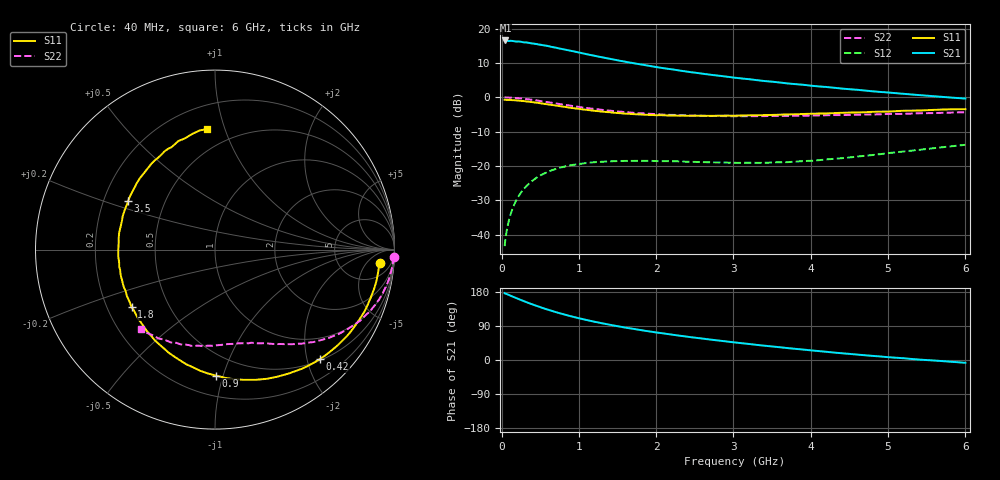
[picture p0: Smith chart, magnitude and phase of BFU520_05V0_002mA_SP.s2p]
! Filename:  P:\Prog\Test\Noise\ATS_data\Testdata_Net\03 Spar\BFU520_APG2013_37_A05_05p0V_002mA_SP_CM01_D.s2p
! Date/Time: Fri 26/Apr/2013 13:00:07
! BFU520_APG2013_37_A05_05p0V_1to20mA_SP_CM01_Bias2_R.s2p
! MDIF S-parameter v. bias file
! BFU520_APG2013_37_A05_05p0V_1to20mA_SP_CM01
! Date/time Tue Apr 23 15:26:19 2013
! VAR V_out= 5.0000
! VAR I_out= 1.9950
! VAR V_in= 0.8075
! VAR I_in= 0.0222
! Device data file deembeded for feedlines and parallel
! Original file: \03 Spar\BFU520_APG2013_37_A05_05p0V_002mA_SP_CM01_R.s2p
! Feed-files: PR047V01_250413_Feed1.s2p, PR047V01_250413_Feed2.s2p
! Parallel-file: PR047V01_250413_Par.s2p
# MHz S MA R 50
!  Freq-MHz  S11-mag  S11-arg  S21-mag  S21-arg  S12-mag  S12-arg  S22-mag  S22-arg
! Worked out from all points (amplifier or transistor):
!   98 points, 40 MHz to 6 GHz, reference 50 ohm
!   highest |S21| = 16.5 dB at 50 MHz (marker M1)
!   |S21| within 3 dB of that: start of sweep to 894.5 MHz
!   unconditionally stable (mu >= 1): 2.993 GHz to 4.97 GHz
!   at 300 MHz: K = 0.11, MSG = 21.2 dB, |S12| = -26.4 dB
!   at 1.6 GHz: K = 0.53, MSG = 14.4 dB, |S12| = -18.5 dB
!   at 6 GHz: K = 0.83, MSG = 6.7 dB, |S12| = -13.8 dB
!   S11 on the Smith chart (normalised r, x): 40 MHz: 13, -12; 420 MHz: 0.53, -2.25; 900 MHz: 0.34, -0.95; 1.8 GHz: 0.30, -0.29; 3.5 GHz: 0.30, +0.24; 6 GHz: 0.36, +0.87
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40  0.9211 -4.6  6.69 176.6  0.006855 86.6  0.996 -2.4
50  0.9193 -5.7  6.709 175.0  0.008572 86.3  0.9963 -2.9
100  0.916 -11.2  6.587 171.2  0.01699 82.9  0.9909 -6.1
120  0.9133 -13.6  6.634 169.4  0.0203 81.6  0.9881 -7.3
180  0.904 -20.3  6.494 164.4  0.03012 77.4  0.979 -11.0
220  0.8961 -24.8  6.479 160.9  0.03632 74.8  0.9696 -13.4
320  0.8721 -35.7  6.284 152.8  0.05091 68.4  0.9437 -19.1
420  0.8452 -46.1  6.03 145.2  0.06382 62.5  0.911 -24.2
600  0.7891 -63.8  5.573 132.8  0.08262 53.2  0.8492 -32.4
700  0.7595 -72.8  5.278 126.5  0.09063 48.6  0.8149 -36.4
900  0.7023 -89.4  4.736 115.3  0.1032 41.2  0.7539 -43.1
1050  0.6671 -100.7  4.362 107.8  0.1092 36.5  0.7115 -47.4
1200  0.6371 -111.2  4.025 101.1  0.1136 32.5  0.6771 -51.1
1450  0.597 -126.8  3.543 91.1  0.118 27.4  0.6316 -56.5
1800  0.5646 -145.3  3.01 79.1  0.1193 22.5  0.586 -62.8
2050  0.5497 -157.2  2.698 71.4  0.1181 20.3  0.5639 -67.2
2500  0.5404 -175.8  2.284 59.0  0.1151 18.9  0.542 -74.5
3100  0.5428 162.6  1.883 44.5  0.1116 21.7  0.5315 -84.0
3500  0.5544 150.8  1.687 35.7  0.1129 25.6  0.5354 -90.4
4100  0.5803 133.7  1.441 23.6  0.1218 32.1  0.5439 -100.4
5200  0.6383 108.6  1.123 4.7  0.1631 38.2  0.575 -119.1
6000  0.6724 93.9  0.9589 -7.4  0.204 36.4  0.6066 -133.1
